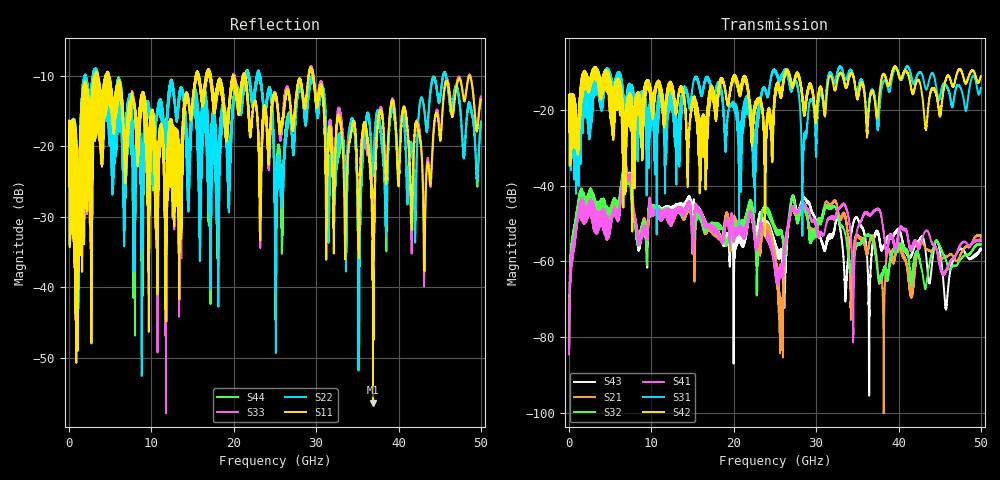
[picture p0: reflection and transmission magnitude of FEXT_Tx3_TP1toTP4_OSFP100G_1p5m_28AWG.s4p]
! Touchstone data
! Created: 27-Feb-2019 by IdEM 12 (12.1.0)
! COMMENTS
!  Created Wed Feb 27 09:43:39 2019
!  64 Port Network Data from SP1.SP block
!  freq  magS1_1  angS1_1  magS1_2  angS1_2  magS1_3  angS1_3  magS1_4  angS1_4
!  magS1_5  angS1_5  magS1_6  angS1_6  magS1_7  angS1_7  magS1_8  angS1_8
!  magS1_9  angS1_9  magS1_10  angS1_10  magS1_11  angS1_11  magS1_12  angS1_12
!  magS1_13  angS1_13  magS1_14  angS1_14  magS1_15  angS1_15  magS1_16  angS1_16
!  magS1_17  angS1_17  magS1_18  angS1_18  magS1_19  angS1_19  magS1_20  angS1_20
!  magS1_21  angS1_21  magS1_22  angS1_22  magS1_23  angS1_23  magS1_24  angS1_24
!  magS1_25  angS1_25  magS1_26  angS1_26  magS1_27  angS1_27  magS1_28  angS1_28
!  magS1_29  angS1_29  magS1_30  angS1_30  magS1_31  angS1_31  magS1_32  angS1_32
!  magS1_33  angS1_33  magS1_34  angS1_34  magS1_35  angS1_35  magS1_36  angS1_36
!  magS1_37  angS1_37  magS1_38  angS1_38  magS1_39  angS1_39  magS1_40  angS1_40
!  magS1_41  angS1_41  magS1_42  angS1_42  magS1_43  angS1_43  magS1_44  angS1_44
!  magS1_45  angS1_45  magS1_46  angS1_46  magS1_47  angS1_47  magS1_48  angS1_48
!  magS1_49  angS1_49  magS1_50  angS1_50  magS1_51  angS1_51  magS1_52  angS1_52
!  magS1_53  angS1_53  magS1_54  angS1_54  magS1_55  angS1_55  magS1_56  angS1_56
!  magS1_57  angS1_57  magS1_58  angS1_58  magS1_59  angS1_59  magS1_60  angS1_60
!  magS1_61  angS1_61  magS1_62  angS1_62  magS1_63  angS1_63  magS1_64  angS1_64
!  magS2_1  angS2_1  magS2_2  angS2_2  magS2_3  angS2_3  magS2_4  angS2_4
!  magS2_5  angS2_5  magS2_6  angS2_6  magS2_7  angS2_7  magS2_8  angS2_8
!  magS2_9  angS2_9  magS2_10  angS2_10  magS2_11  angS2_11  magS2_12  angS2_12
!  magS2_13  angS2_13  magS2_14  angS2_14  magS2_15  angS2_15  magS2_16  angS2_16
!  magS2_17  angS2_17  magS2_18  angS2_18  magS2_19  angS2_19  magS2_20  angS2_20
!  magS2_21  angS2_21  magS2_22  angS2_22  magS2_23  angS2_23  magS2_24  angS2_24
!  magS2_25  angS2_25  magS2_26  angS2_26  magS2_27  angS2_27  magS2_28  angS2_28
!  magS2_29  angS2_29  magS2_30  angS2_30  magS2_31  angS2_31  magS2_32  angS2_32
!  magS2_33  angS2_33  magS2_34  angS2_34  magS2_35  angS2_35  magS2_36  angS2_36
!  magS2_37  angS2_37  magS2_38  angS2_38  magS2_39  angS2_39  magS2_40  angS2_40
!  magS2_41  angS2_41  magS2_42  angS2_42  magS2_43  angS2_43  magS2_44  angS2_44
!  magS2_45  angS2_45  magS2_46  angS2_46  magS2_47  angS2_47  magS2_48  angS2_48
!  magS2_49  angS2_49  magS2_50  angS2_50  magS2_51  angS2_51  magS2_52  angS2_52
!  magS2_53  angS2_53  magS2_54  angS2_54  magS2_55  angS2_55  magS2_56  angS2_56
!  magS2_57  angS2_57  magS2_58  angS2_58  magS2_59  angS2_59  magS2_60  angS2_60
!  magS2_61  angS2_61  magS2_62  angS2_62  magS2_63  angS2_63  magS2_64  angS2_64
!  magS3_1  angS3_1  magS3_2  angS3_2  magS3_3  angS3_3  magS3_4  angS3_4
!  magS3_5  angS3_5  magS3_6  angS3_6  magS3_7  angS3_7  magS3_8  angS3_8
!  magS3_9  angS3_9  magS3_10  angS3_10  magS3_11  angS3_11  magS3_12  angS3_12
!  magS3_13  angS3_13  magS3_14  angS3_14  magS3_15  angS3_15  magS3_16  angS3_16
!  magS3_17  angS3_17  magS3_18  angS3_18  magS3_19  angS3_19  magS3_20  angS3_20
!  magS3_21  angS3_21  magS3_22  angS3_22  magS3_23  angS3_23  magS3_24  angS3_24
!  magS3_25  angS3_25  magS3_26  angS3_26  magS3_27  angS3_27  magS3_28  angS3_28
!  magS3_29  angS3_29  magS3_30  angS3_30  magS3_31  angS3_31  magS3_32  angS3_32
!  magS3_33  angS3_33  magS3_34  angS3_34  magS3_35  angS3_35  magS3_36  angS3_36
!  magS3_37  angS3_37  magS3_38  angS3_38  magS3_39  angS3_39  magS3_40  angS3_40
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# Hz S MA R 50
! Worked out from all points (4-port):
!   5000 points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, 10 MHz to 50 GHz, reference 50 ohm
!   strongest paths, dB at 10 MHz, 12.51 GHz, 25.01 GHz, 37.51 GHz, 50 GHz:
!     S42: -19.6, -14.6, -15.6, -20.4, -11.1
!     S31: -19.6, -16.6, -9.8, -25.4, -14.2
!     S41: -84.6, -47.4, -62.9, -46.1, -54.6
!     S32: -81.0, -47.7, -51.1, -63.9, -55.7
!     S21: -83.1, -47.8, -59.9, -62.9, -53.5
!     S43: -82.9, -46.7, -55.6, -52.2, -56.9
!   lowest |S11| = -56.3 dB at 36.9 GHz (marker M1), VSWR 1.00, Z = 50.1 + j0.121 ohm
!   |S11| at or under -10 dB: 4.861 GHz to 15.4 GHz (10.54 GHz wide, 104 % of centre); 21.38 GHz to 29.07 GHz (7.682 GHz wide, 30.5 % of centre); 29.66 GHz to end of sweep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
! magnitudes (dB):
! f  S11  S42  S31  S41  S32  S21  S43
! 10 MHz  -19.1  -19.6  -19.6  -84.6  -81.0  -83.1  -82.9
! 1.26 GHz  -34.3  -25.0  -31.8  -45.0  -42.0  -43.8  -43.6
! 6.75 GHz  -23.7  -28.5  -24.7  -34.8  -33.7  -34.3  -34.1
! 25.74 GHz  -17.8  -14.9  -11.0  -61.8  -52.7  -74.5  -58.7
! 27.1 GHz  -16.7  -14.1  -14.6  -45.5  -42.9  -45.9  -43.1
! 36.9 GHz  -56.3  -15.2  -14.9  -46.9  -54.9  -53.5  -55.0
! 50 GHz  -13.4  -11.1  -14.2  -54.6  -55.7  -53.5  -56.9
